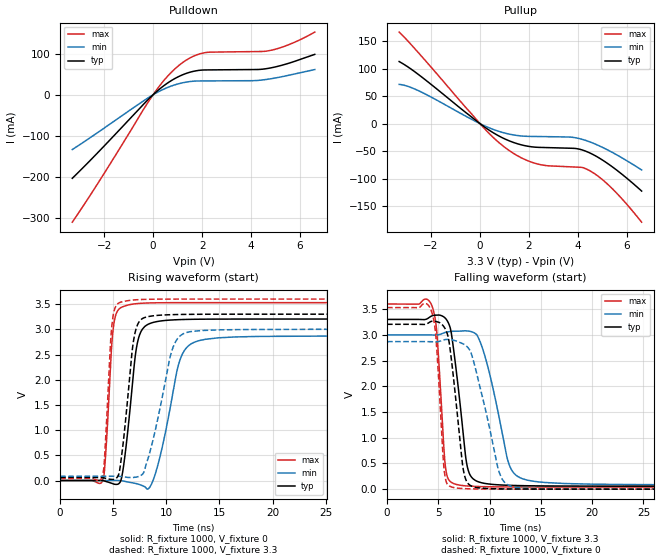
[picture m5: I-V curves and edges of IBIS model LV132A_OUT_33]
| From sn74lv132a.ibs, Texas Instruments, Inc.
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[Model]   LV132A_OUT_33
Model_type  Output
Vref =   0
Rref =   1000
Cref =   50p
Vmeas =   1.65
| variable   typ   min   max
C_comp   7.26pF   3.48pF   16.96pF
| C_pullup   5.52pF   3.48pF   7.55pF
| C_pulldown   9.00pF   4.04pF   16.96pF
[Temperature Range]   40   100   -40
| Ambient temperature   25   85   -40
[Voltage range]   3.3   3   3.6
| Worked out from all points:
|   slope of the pulldown table from 0 to 0.495 V, typ, clamps not added: 20.1 ohm
|   slope of the pullup table from 0 to 0.495 V, typ, clamps not added: 32.2 ohm
|   rising waveform, R_fixture 1000, V_fixture 0: 20-80 % time 948ps typ, 1.63ns min, 565ps max; typ from 0 V to 3.2 V
|   falling waveform, R_fixture 1000, V_fixture 3.3: 20-80 % time 1.09ns typ, 1.87ns min, 649ps max; typ from 3.3 V to 0.059 V
|   rising waveform, R_fixture 1000, V_fixture 3.3: 20-80 % time 913ps typ, 1.74ns min, 532ps max; typ from 0.059 V to 3.3 V
|   falling waveform, R_fixture 1000, V_fixture 0: 20-80 % time 1.02ns typ, 1.95ns min, 627ps max; typ from 3.21 V to 0 V
[Pulldown]
| LV132A_OUT_33
|   Voltage   I(typ)   I(min)   I(max)
-3.3V     -204.2mA   -134mA     -311.5mA
-2.13V    -133.5mA   -86.93mA   -204.7mA
-405mV    -24.2mA    -15.57mA   -37.07mA
-15mV     -843.8uA   -535uA     -1.311mA
545mV     26.72mA    16.58mA    42.11mA
1.105V    46.16mA    27.83mA    74.1mA
1.62V     56.84mA    32.96mA    93.4mA
2.13V     60.6mA     33.75mA    102.9mA
4.12V     61.59mA    34.47mA    105.5mA
4.89V     66.68mA    39.88mA    109.7mA
5.69V     79.84mA    49.61mA    126mA
6.6V      98.63mA    61.55mA    153.1mA
[Pullup]
| LV132A_OUT_33
|   Voltage   I(typ)   I(min)   I(max)
-3.3V     113.1mA    71.46mA    166.7mA
-2.42V    86.27mA    58.02mA    124.4mA
135mV     -4.526mA   -2.94mA    -6.758mA
955mV     -26.64mA   -16.52mA   -41.15mA
1.615V    -37.78mA   -22.16mA   -60.56mA
2.27V     -42.95mA   -23.43mA   -72.52mA
3.895V    -45.24mA   -25.73mA   -79.13mA
4.19V     -48.2mA    -28.85mA   -80.05mA
4.485V    -53.45mA   -33.27mA   -85.86mA
4.92V     -64.07mA   -41.53mA   -99.11mA
5.41V     -78.93mA   -52.61mA   -118.8mA
6.6V      -122.8mA   -84.42mA   -179.5mA
[Ramp]
| LV132A_OUT_33
| variable   typ   min   max
dV/dt_r   1.97/9.74E-10   1.82/1.74E-09   2.15/5.78E-10
dV/dt_f   2.00/1.13E-09   1.80/1.93E-09   2.19/6.76E-10
R_load = 1000
[Rising Waveform]
| LV132A_OUT_33
R_fixture =   1000
C_fixture =   0
L_fixture =   0
V_fixture =   0
V_fixture_min = 0
V_fixture_max = 0
|   Time   V(typ)   V(min)   V(max)
0s        1.651nV    7.495nV    1.082nV
4.02ns    -1.798mV   -3.346uV   7.824mV
4.275ns   -16.42mV   79.96uV    485.2mV
5.01ns    -66.88mV   1.566mV    3.033V
6.11ns    505.3mV    -17.27mV   3.464V
7.27ns    2.724V     -66.39mV   3.51V
8.695ns   3.133V     -26.47mV   3.525V
11.22ns   3.192V     2.354V     3.529V
12.86ns   3.2V       2.761V     3.529V
50ns      3.204V     2.866V     3.529V
[Falling Waveform]
| LV132A_OUT_33
R_fixture =   1000
C_fixture =   0
L_fixture =   0
V_fixture =   3.3
V_fixture_min = 3
V_fixture_max = 3.6
|   Time   V(typ)   V(min)   V(max)
0s        3.3V       3V         3.6V
4.395ns   3.371V     2.998V     3.557V
4.85ns    3.384V     2.998V     3.057V
5.695ns   3.321V     3.048V     439mV
6.58ns    2.58V      3.071V     103.1mV
8.1ns     275.4mV    3.068V     58.19mV
9.54ns    111.6mV    2.592V     48.16mV
11.9ns    74.84mV    480.1mV    43.12mV
13.26ns   68.13mV    199.3mV    42.14mV
50ns      58.57mV    83.94mV    41.16mV
[Rising Waveform]
| LV132A_OUT_33
R_fixture =   1000
C_fixture =   0
L_fixture =   0
V_fixture =   3.3
V_fixture_min = 3
V_fixture_max = 3.6
|   Time   V(typ)   V(min)   V(max)
0s        58.57mV    83.92mV    41.16mV
3.95ns    58.54mV    83.93mV    64.57mV
4.17ns    49.91mV    83.99mV    405.1mV
4.885ns   21.01mV    85.11mV    3.099V
5.705ns   357.5mV    81.01mV    3.539V
6.93ns    2.796V     61.93mV    3.582V
8.01ns    3.237V     251mV      3.594V
10.5ns    3.29V      2.557V     3.599V
11.88ns   3.296V     2.935V     3.6V
50ns      3.3V       3V         3.6V
[Falling Waveform]
| LV132A_OUT_33
R_fixture =   1000
C_fixture =   0
L_fixture =   0
V_fixture =   0
V_fixture_min = 0
V_fixture_max = 0
|   Time   V(typ)   V(min)   V(max)
0s        3.205V     2.868V     3.53V
4.32ns    3.262V     2.867V     3.466V
4.765ns   3.26V      2.866V     2.959V
5.575ns   3.15V      2.904V     369mV
6.26ns    2.549V     2.905V     44.76mV
7.355ns   491.4mV    2.831V     12.39mV
7.725ns   166.8mV    2.786V     9.044mV
10.92ns   6.626mV    344.2mV    1.19mV
12.08ns   3.871mV    58.12mV    642.5uV
50ns      177.6nV    2.848uV    94.39nV
